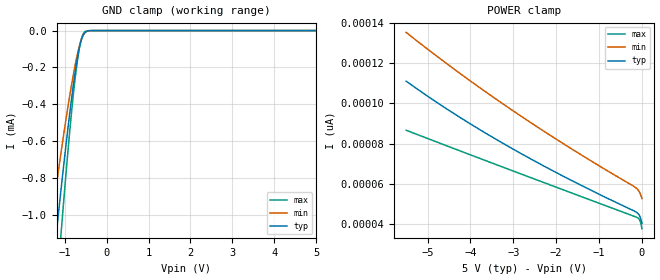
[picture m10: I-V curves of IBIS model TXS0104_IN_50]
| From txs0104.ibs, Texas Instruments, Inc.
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[Model]   TXS0104_IN_50
Model_type  Input
Vinl=1.35
Vinh=3.85
| variable   typ   min   max
C_comp   0.21pF   0.16pF   0.25pF
[Temperature Range]   40   100   -40
| Ambient temperature   25   85   -40
[Voltage range]   5   4.5   5.5
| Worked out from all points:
|   GND clamp passes 1 mA (typ) near -1.16 V on its own axis
[GND Clamp]
| TXS0104_IN_50
|   Voltage   I(typ)   I(min)   I(max)
-5.5V     -12.44mA   -9.732mA   -15.69mA
-1.375V   -1.484mA   -1.129mA   -1.928mA
-1.32V    -1.359mA   -1.035mA   -1.763mA
-1.19V    -1.071mA   -818.2uA   -1.381mA
-1.095V   -868.2uA   -666.1uA   -1.11mA
-1.075V   -826.4uA   -634.8uA   -1.054mA
-855mV    -395.3uA   -313.4uA   -475.6uA
-740mV    -203.5uA   -170.5uA   -230.9uA
-670mV    -110.5uA   -98.45uA   -117.1uA
-620mV    -61.6uA    -57.47uA   -57.78uA
-510mV    -8.88uA    -9.112uA   -4.52uA
5V        40.56pA    62.64pA    30.05pA
[POWER Clamp]
| TXS0104_IN_50
|   Voltage   I(typ)   I(min)   I(max)
-5.5V     111pA      135.2pA    86.62pA
-4.94V    102.7pA    125.9pA    82.04pA
-4.345V   94.35pA    116.4pA    77.2pA
-3.085V   78.22pA    97.41pA    67.04pA
-1.735V   62.71pA    78.62pA    56.24pA
-135mV    46pA       57.93pA    43.51pA
-85mV     45.11pA    56.82pA    42.92pA
-50mV     43.87pA    55.53pA    41.93pA
-25mV     42.42pA    54.24pA    40.32pA
-95.1fV   40.56pA    52.72pA    37.78pA
